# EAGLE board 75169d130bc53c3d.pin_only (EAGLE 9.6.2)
REV: B

Size 38.1 x 33.02 mm. Coordinates in mm from the lower left corner, seen from the top.
Outline: 0,30.48 0,2.54 arc90 2.54,0 35.56,0 arc90 38.1,2.54 38.1,30.48 arc90 35.56,33.02 2.54,33.02 arc90 0,30.48
Copper layers (1*16): Top 0.035mm / dielectric 1.5mm / Bottom 0.035mm
Design rules "adafruit 7-7": minimum track width 6mil, minimum drill 15.5mil, track to track 8mil, track to pad 7mil, pad to pad 7mil, via to via 7mil, smd to smd 7mil, copper to edge 10mil, drill to drill 8mil, minimum pad ring 10mil, minimum via ring 8mil, stop-mask expansion 2mil, vias tented up to drill 20mil, thermal gap 10mil
Net classes: 1 highpower: width 0.305 mm, drill 0.483 mm

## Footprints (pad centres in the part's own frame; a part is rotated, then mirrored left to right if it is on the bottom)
SOLDERJUMPER_ARROW_NOPASTE = smd 0.762 x 1.524: 1 -1.016,0; 2 1.016,0
SOLDERJUMPER_CLOSEDWIRE = smd 1.168 x 1.6: 1 -0.762,0; 2 0.762,0 | smd 0.635 x 0.203: WIRE 0,0
JST-PH-2-SMT-RA = smd 1 x 4.6: 1 1,-3.7; 2 -1,-3.7 | smd 1.6 x 3.4: NC1 -3.4,1.5; NC2 3.4,1.5
0805-NO = smd 1.24 x 1.5: 1 -0.95,0; 2 0.95,0
CHIPLED_0603 = smd 0.8 x 0.8: A 0,-0.75; C 0,0.75
SMADIODE = smd 1.778 x 2.159: A 2.019,0; C -2.045,0
FIDUCIAL_1MM = smd 1 x 1: 1 0,0
1X02_ROUND = drill 1 pad 1.778: 1 -1.27,0; 2 1.27,0
1X01_OVAL = drill 1 pad 1.676 long: 1 0,0
1X11_ROUND_76 = drill 1 pad 1.93: 1 -12.7,0; 2 -10.16,0; 3 -7.62,0; 4 -5.08,0; 5 -2.54,0; 6 0,0; 7 2.54,0; 8 5.08,0; 9 7.62,0; 10 10.16,0; 11 12.7,0
0603-NO = smd 1.075 x 1: 1 -0.85,0; 2 0.85,0
SOLDERJUMPER_2WAY_OPEN_NOPASTE = smd 1.168 x 1.6: 1 -1.397,0; 2 0,0; 3 1.397,0
MOUNTINGHOLE_2.5_PLATED = drill 2.5 pad 3.2: P$1 0,0
USB_C_CUSB31-CFM2AX-01-X = smd 0.575 x 1.15: A1B12 -3.2,3.545; A4B9 -2.4,3.545; B1A12 3.2,3.545; B4A9 2.4,3.545 | smd 0.275 x 1.15: A5 -1.25,3.545; A6 -0.25,3.545; A7 0.25,3.545; A8 1.25,3.545; B5 1.75,3.545; B6 0.75,3.545; B7 -0.75,3.545; B8 -1.75,3.545 | drill 0.6 pad 1 long: M1 -4.32,2.97; M2 4.32,2.97; M3 -4.32,-1.21; M4 4.32,-1.21 | hole 0.65: 2.89,2.47; -2.89,2.47
DCJACK_2MM_SMT = smd 2.4 x 2: 1 0,5.5; 1' 6.2,5.5; 2 0,-5.5; 3 6.2,-5.5 | hole 1.6: 0,0 | hole 1.8: 4.5,0
QFN16_3MM = smd 0.8 x 0.28: 1 -1.5,0.75; 2 -1.5,0.25; 3 -1.5,-0.25; 4 -1.5,-0.75; 9 1.5,-0.75; 10 1.5,-0.25; 11 1.5,0.25; 12 1.5,0.75 | smd 0.28 x 0.8: 5 -0.75,-1.5; 6 -0.25,-1.5; 7 0.25,-1.5; 8 0.75,-1.5; 13 0.75,1.5; 14 0.25,1.5; 15 -0.25,1.5; 16 -0.75,1.5 | smd 1.5 x 1.5: THERMAL 0,0

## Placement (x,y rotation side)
0.5A  [SOLDERJUMPER_ARROW_NOPASTE]  20.57,6.35 180 top
1.5A  [SOLDERJUMPER_ARROW_NOPASTE]  20.57,10.79 180 top
1A  [SOLDERJUMPER_CLOSEDWIRE]  20.57,8.64 180 top
BATT  JST 2PH  [JST-PH-2-SMT-RA]  34.54,10.79 270 top
C1  10uF  [0805-NO]  13.72,11.05 180 top
C2  10uF  [0805-NO]  20.83,19.18 180 top
C3  10uF  [0805-NO]  25.53,22.35 90 top
C4  10uF  [0805-NO]  27.43,22.35 90 top
C5  10uF  [0805-NO]  27.3,7.24 270 top
C6  10uF  [0805-NO]  27.3,10.79 90 top
C9  10uF  [0805-NO]  13.97,16.13 180 top
D1  GREEN  [CHIPLED_0603]  32.38,15.75 90 top
D2  SK34A  [SMADIODE]  12.19,13.59 180 top
D3  RED  [CHIPLED_0603]  32.38,17.27 90 top
D4  SK34A  [SMADIODE]  13.84,20.57 90 top
FID1  FIDUCIAL_1MM  [FIDUCIAL_1MM]  13.34,25.78 0 top
FID2  FIDUCIAL_1MM  [FIDUCIAL_1MM]  32.77,31.88 0 top
FID3  FIDUCIAL_1MM  [FIDUCIAL_1MM]  4.32,16.13 0 top
JP1  [1X02_ROUND]  10.16,9.4 0 top
JP2  [1X01_OVAL]  22.73,24.38 0 top
JP3  [1X11_ROUND_76]  19.05,2.54 180 top
JP4  [1X01_OVAL]  17.65,24.38 0 top
R1  1K  [0603-NO]  17.53,18.16 180 top
R2  10K  [0603-NO]  17.78,15.11 180 top
R3  590  [0603-NO]  17.91,12.32 270 top
R4  5.1K  [0603-NO]  9.91,7.62 180 top
R5  2K  [0603-NO]  17.91,6.22 270 top
R6  5.1K  [0603-NO]  10.16,11.43 180 top
R7  10K  [0603-NO]  26.29,18.54 0 top
R8  10K  [0603-NO]  26.42,13.59 0 top
R9  1K  [0603-NO]  17.91,9.27 90 top
R10  10K  [0603-NO]  16.26,8.89 90 top
R11  10K  [0603-NO]  26.29,16.89 0 top
SJ1  [SOLDERJUMPER_2WAY_OPEN_NOPASTE]  27.3,13.97 0 bottom
SJ2  [SOLDERJUMPER_2WAY_OPEN_NOPASTE]  27.3,16.26 0 bottom
SYSOUT  JST 2PH  [JST-PH-2-SMT-RA]  34.54,22.23 270 top
THERM  [SOLDERJUMPER_CLOSEDWIRE]  15.37,6.35 180 top
U$3  MOUNTINGHOLE2.5  [MOUNTINGHOLE_2.5_PLATED]  2.54,2.54 0 top
U$4  MOUNTINGHOLE2.5  [MOUNTINGHOLE_2.5_PLATED]  2.54,30.48 0 top
U$11  MOUNTINGHOLE2.5  [MOUNTINGHOLE_2.5_PLATED]  35.56,30.48 0 top
U$12  MOUNTINGHOLE2.5  [MOUNTINGHOLE_2.5_PLATED]  35.56,2.54 0 top
U$14  [ADAFRUIT_5MM]  25.15,24 0 top
U$18  [PCBFEAT-REV-040]  36.32,27.05 0 bottom
X2  USB Type C  [USB_C_CUSB31-CFM2AX-01-X]  2.79,10.16 270 top
X3  2.1mm DC  [DCJACK_2MM_SMT]  1.78,21.72 0 top
X4  BQ24074  [QFN16_3MM]  21.59,15.88 90 top

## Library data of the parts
0.5A 1.5A FID1-FID3 U$3 U$4 U$11 U$12 = microbuilder; BOM: EXCLUDE
1A C1-C6 C9 D1-D4 JP1-JP4 R1-R11 SJ1 SJ2 THERM U$14 U$18 X2 X3 = microbuilder
BATT SYSOUT = adafruit
X4 = adafruit_power

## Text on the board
tPlace: 1.5A USB/DC/Solar / LiPo Charger | 10V Max | Load Out | Opt. Cap | CHG | GOOD | 1.5A | THM | 1.0A | 0.5A | LiPo Batt | VBUS | THERM | CE | CHG | GND | GND | GND | ISET | PGOOD | OUT | LIPO
bPlace: 0.5A~1.5A USB/DC/Solar / LiPo Charger with Load / Sharing Output (bq24074) | Load Output is shared with DC/USB / input priority & regulated to 4.4V or less | EN1 | Solar/DC In is 10V Max | Low | High | EN2 | Use any 3.7/4.2V LiPoly/LiIon | D+ | D-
